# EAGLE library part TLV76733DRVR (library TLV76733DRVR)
Adjustable and fixed 1-A 16-V positive-voltage low-dropout (LDO) linear regulator Source: Datasheet
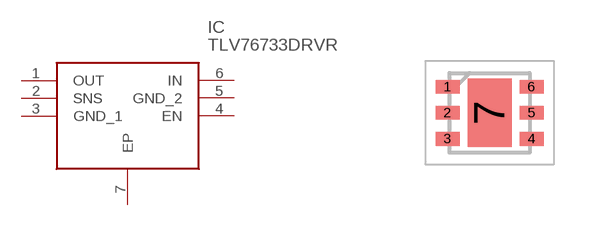
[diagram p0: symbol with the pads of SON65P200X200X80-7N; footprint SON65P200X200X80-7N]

Designator prefix IC

## TLV76733DRVR (Description: Adjustable and fixed 1-A 16-V positive-voltage low-dropout (LDO) linear regulator; Height: 0.8mm; Manufacturer_Name: Texas Instruments; Manufacturer_Part_Number: TLV76733DRVR; Mouser_Part_Number: 595-TLV76733DRVR; Mouser_Price-Stock: https://www.mouser.co.uk/ProductDetail/Texas-Instruments/TLV76733DRVR?qs=9r4v7xj2LnmGIkwTuPlHig%3D%3D)  [SON65P200X200X80-7N]
1  OUT
2  SNS
3  GND_1
4  EN
5  GND_2
6  IN
7  EP

## Footprint SON65P200X200X80-7N (pad centres in mm)
DRV0006A
smd 0.6 x 0.35: 1 -1.05,0.65; 2 -1.05,0; 3 -1.05,-0.65; 4 1.05,-0.65; 5 1.05,0; 6 1.05,0.65
smd 1.1 x 1.7: 7 0,0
